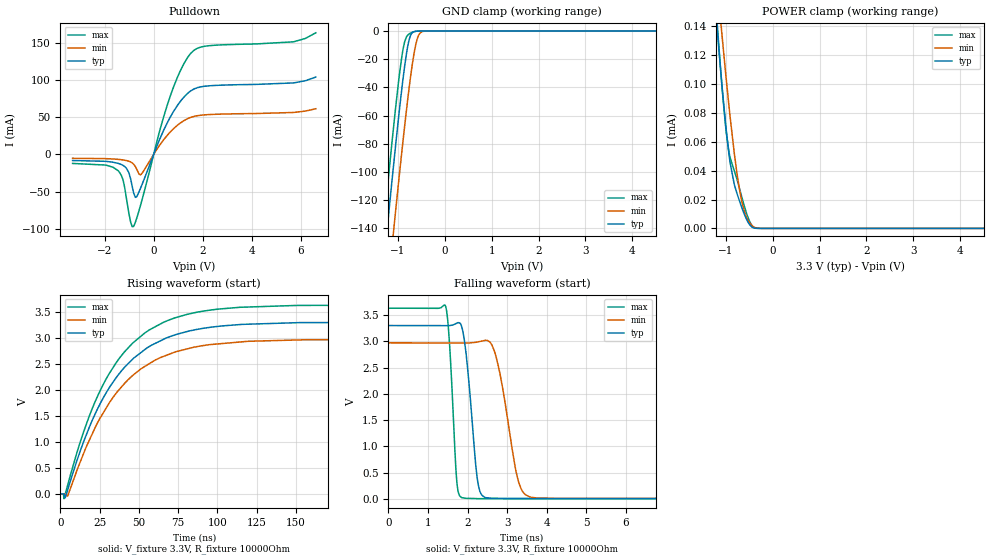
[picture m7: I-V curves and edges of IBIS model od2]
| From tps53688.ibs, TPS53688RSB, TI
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|   od2 Model
[Model]   od2
Model_type   Open_drain
Polarity   Non-Inverting
Vmeas = 1.65
Vref = 3.3
Cref = 2pF
Rref = 1000
|   typ   min   max
C_comp   1.498pF   1.478pF   1.526pF
[Voltage Range]   3.3   2.97   3.63
|Junction Temperature
[Temperature Range]   25   125   -40
[Pullup Reference]   3.3   2.97   3.63
[Pulldown Reference]   -0   -0   0
[Power Clamp Reference]   3.3   2.97   3.63
[GND Clamp Reference]   0   0   0
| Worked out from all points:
|   slope of the pulldown table from 0 to 0.495 V, typ, clamps not added: 12.8 ohm
|   GND clamp passes 1 mA (typ) near -0.68 V on its own axis
|   falling waveform, V_fixture 3.3V, R_fixture 10000Ohm: 20-80 % time 224ps typ, 385ps min, 145ps max; typ from 3.3 V to 0.004 V
|   rising waveform, V_fixture 3.3V, R_fixture 10000Ohm: 20-80 % time 37.3ns typ, 37.8ns min, 36.5ns max; typ from 0.004 V to 3.3 V
[Pulldown]
|   Voltage   I(typ)   I(min)   I(max)
-3.3V     -8.174mA   -5.195mA   -12.1mA
-1.439V   -12.09mA   -6.65mA    -22.04mA
-1.231V   -15.05mA   -7.476mA   -36.5mA
-1.023V   -23.65mA   -8.991mA   -76.48mA
-815.1mV  -51.84mA   -13.14mA   -96.88mA
-696.3mV  -57.1mA    -19.41mA   -86.56mA
-518.1mV  -44.1mA    -27mA      -66.43mA
570.9mV   43.65mA    26.36mA    68.11mA
1.105V    72.13mA    42.74mA    113.9mA
1.521V    85.78mA    50.01mA    136.4mA
5.689V    96.2mA     56.46mA    151.5mA
6.6V      104.1mA    61.46mA    163.6mA
[GND Clamp]
|   Voltage   I(typ)   I(min)   I(max)
-3.3V     -887.9mA   -924.8mA   -869mA
-1.32V    -172.6mA   -219.1mA   -145.5mA
-1.241V   -145.5mA   -192.3mA   -118.3mA
-1.122V   -105.8mA   -152.6mA   -78.63mA
-1.053V   -83.36mA   -129.9mA   -56.6mA
-953.7mV  -52.71mA   -98.24mA   -28.03mA
-884.4mV  -33.03mA   -76.82mA   -12.4mA
-785.4mV  -10.51mA   -47.95mA   -2.867mA
-696.3mV  -1.441mA   -25.14mA   -944.4uA
-577.5mV  -74.1uA    -4.896mA   -91.01uA
-419.1mV  -1.115uA   -82.31uA   -723.6nA
6.6V      0A         0A         0A
[POWER Clamp]
|   Voltage   I(typ)   I(min)   I(max)
-3.3V     1.047mA    986.4uA    1.182mA
-1.221V   153.9uA    185uA      160.1uA
-1.122V   115.2uA    149.4uA    116.3uA
-1.092V   104.1uA    139uA      104uA
-1.003V   72.97uA    108.5uA    71.39uA
-933.9mV  52.54uA    86.12uA    53.76uA
-815.1mV  30.27uA    51.79uA    39.83uA
-716.1mV  20.07uA    29.05uA    29.01uA
-597.3mV  9.438uA    11.53uA    14.9uA
-498.3mV  2.986uA    4.346uA    5.533uA
-409.2mV  416.4nA    1.171uA    918.5nA
6.6V      0A         0A         0A
[Ramp]
R_load = 10000
|   typ   min   max
dV/dt_r   1.97776/3.71595e-08   1.77872/3.78104e-08   2.1764/3.64491e-08
dV/dt_f   1.97776/2.23816e-10   1.77872/3.8485e-10   2.1764/1.44847e-10
[Falling Waveform]
V_fixture = 3.3V
V_fixture_min = 2.97V
V_fixture_max = 3.63V
R_fixture = 10000Ohm
C_fixture = 0F
|   Time   V(typ)   V(min)   V(max)
0s        3.3V       2.97V      3.63V
1.444ns   3.298V     2.969V     3.673V
1.548ns   3.299V     2.969V     2.923V
1.725ns   3.343V     2.968V     370.3mV
1.827ns   3.329V     2.968V     38.93mV
2.268ns   284.7mV    2.989V     3.905mV
2.699ns   9.979mV    2.764V     3.904mV
3.352ns   5.504mV    195mV      3.903mV
4.273ns   5.5mV      8.295mV    3.9mV
500ns     3.727mV    5.46mV     2.659mV
[Rising Waveform]
V_fixture = 3.3V
V_fixture_min = 2.97V
V_fixture_max = 3.63V
R_fixture = 10000Ohm
C_fixture = 0F
|   Time   V(typ)   V(min)   V(max)
0s        3.727mV    5.46mV     2.659mV
2.253ns   4.157mV    5.648mV    -88.45mV
3.006ns   -72.79mV   5.711mV    -5.577mV
4.561ns   76.88mV    -37.05mV   167.4mV
20.3ns    1.418V     1.158V     1.645V
35.62ns   2.238V     1.94V      2.526V
53.81ns   2.774V     2.45V      3.093V
80.8ns    3.12V      2.787V     3.45V
156.6ns   3.291V     2.962V     3.621V
500ns     3.3V       2.97V      3.63V
